[IBIS Ver]   4.0
[Comment Char] |_char
[File name]   pse84_wlb154.ibs
[File Rev] 1.2
[Date] 10/27/2023
[Source] Infineon Technologies IBIS team
[Notes]
|Rev. 1.0 - Initial model 12/8/2021
|Rev. 1.1 - Update with RLC 8/17/2023
|Rev. 1.2 - Included pins for MIPI-DPHY DSI and USB 10/23/2023
|Supports 1.8 V IO Interface and 3.3 V RF Switch Control Interface.
|The temperature range is -40 to 125C.
|This model was syntax checked with Hyperlynx 4.2 visual IBIS
|editor and ibischk7_64 IBIS checker.
|There were 0 syntax errors.
[Disclaimer]   The model given below represents a 220-pin package.
[Copyright]   (C) COPYRIGHT 2023, Infineon Technologies AG.
[Component] PSOCE84
[Manufacturer] Infineon Technologies AG
| Package model WLBGA154 was extracted from simulation tool.
[Package]
|   typ   min   max
R_pkg   0.37778   0.02885   0.99963
L_pkg   0.755n   0.113n   1.94n
C_pkg   0.272p   0.0783p   0.61p
[Pin]   Signal_name   model_name   R_pin   L_pin   C_pin
|L5   DSI_CLK_N_PAD   PAD   0.18036 3.56E-10   1.32E-13
|L4   DSI_CLK_P_PAD   PAD   0.22925 5.05E-10   1.68E-13
|J5   DSI_DATA0_N_PAD PAD   0.34681 7.02E-10   1.90E-13
|H5   DSI_DATA0_P_PAD PAD   0.32737 6.89E-10   1.82E-13
|H4   DSI_DATA1_N_PAD PAD   0.35927 7.29E-10   1.94E-13
|J4   DSI_DATA1_P_PAD PAD   0.34002 6.83E-10   1.82E-13
|G5   DSI_REXT_PAD   PAD   0.17871 5.97E-10   3.09E-13
G4   P12_0_PAD   1p8_ioi2c_wbso_h   0.58601 1.03E-09   3.09E-13
F5   P12_1_PAD   1p8_ioi2c_wbso_h   0.66384 1.24E-09   3.42E-13
F6   P12_2_PAD   1p8_ioi2c_wbso_h   0.76369 1.39E-09   4.00E-13
F7   P12_3_PAD   1p8_ioi2c_wbso_h   0.81887 1.50E-09   4.18E-13
F8   P12_4_PAD   1p8_ioi2c_wbso_h   0.93099 1.68E-09   5.32E-13
F9   P12_5_PAD   1p8_ioi2c_wbso_h   0.99963 1.80E-09   5.79E-13
G14   P13_0_PAD   1p8_gpib_3swbso_h   0.065427 1.91E-10   1.40E-13
J14   P13_1_PAD   1p8_ioi2c_wbso_h   0.29198 5.62E-10   1.54E-13
F14   P13_2_PAD   1p8_ioi2c_wbso_h   0.028854 1.35E-10   1.02E-13
K14   P13_3_PAD   1p8_ioi2c_wbso_h   0.39961 7.26E-10   3.44E-13
K13   P13_4_PAD   1p8_ioi2c_wbso_h   0.42314 7.99E-10   3.99E-13
E14   P13_5_PAD   1p8_gpib_3swbso_h   0.042433 1.13E-10   2.05E-13
G13   P14_3_PAD   1p8_ioi2c_wbso_h   0.32481 6.11E-10   2.16E-13
J13   P14_4_PAD   1p8_ioi2c_wbso_h   0.4981  8.90E-10   2.78E-13
C14   P15_0_PAD   1p8_ioi2c_wbso_h   0.14092 3.40E-10   1.43E-13
B14   P15_1_PAD   1p8_ioi2c_wbso_h   0.050643 2.09E-10   1.07E-13
G12   P15_2_PAD   1p8_ioi2c_wbso_h   0.55579 1.00E-09   4.33E-13
D13   P15_3_PAD   1p8_ioi2c_wbso_h   0.27529 5.42E-10   1.89E-13
J12   P16_0_PAD   3p3_gpio_wbso_h 0.77613 1.26E-09   5.75E-13
H11   P16_1_PAD   3p3_gpio_wbso_h 0.6983  1.20E-09   4.40E-13
A12   P16_2_PAD   3p3_gpio_wbso_h 0.039971   1.63E-10   9.91E-14
G11   P16_3_PAD   3p3_gpio_wbso_h 0.62882 1.11E-09   3.34E-13
F11   P16_4_PAD   3p3_gpio_wbso_h 0.53345 9.60E-10   3.01E-13
E11   P16_5_PAD   3p3_gpio_wbso_h 0.43008 8.36E-10   2.56E-13
D11   P16_6_PAD   3p3_gpio_wbso_h 0.31519 7.16E-10   2.19E-13
A11   P16_7_PAD   3p3_gpio_wbso_h 0.064   2.05E-10   1.16E-13
G10   P17_0_PAD   3p3_gpio_wbso_h 0.57169 1.07E-09   4.73E-13
F10   P17_1_PAD   3p3_gpio_wbso_h 0.51457 9.91E-10   2.90E-13
E10   P17_2_PAD   3p3_gpio_wbso_h 0.40617 8.30E-10   2.58E-13
E9   P17_3_PAD   3p3_gpio_wbso_h 0.42474 8.38E-10   2.51E-13
D10   P17_4_PAD   3p3_gpio_wbso_h 0.36553 7.76E-10   2.34E-13
D9   P17_5_PAD   3p3_gpio_wbso_h 0.36885 7.43E-10   2.30E-13
C10   P17_6_PAD   3p3_gpio_wbso_h 0.31893 7.04E-10   2.20E-13
H7   P18_0_PAD   1p8_gpib_3swbso_h   0.35662 6.76E-10   2.25E-13
J7   P18_1_PAD   1p8_gpib_3swbso_h   0.25345 4.81E-10   1.87E-13
G8   P19_0_PAD   1p8_gpib_3swbso_h   0.44499 8.18E-10   2.58E-13
H8   P19_1_PAD   1p8_gpib_3swbso_h   0.35458 6.30E-10   2.94E-13
A10   P2_0_PAD   1p8_hsio_wbso_h   0.53479 1.94E-09   6.10E-13
F4   P21_0_PAD   1p8_ioi2c_wbso_h   0.62566 1.14E-09   3.26E-13
E6   P21_1_PAD   1p8_ioi2c_wbso_h   0.67341 1.49E-09   5.08E-13
E5   P21_2_PAD   1p8_ioi2c_wbso_h   0.71959 1.27E-09   5.11E-13
E4   P21_3_PAD   1p8_ioi2c_wbso_h   0.69725 1.16E-09   4.87E-13
D6   P21_7_PAD   1p8_ioi2c_wbso_h   0.54873 1.61E-09   4.24E-13
E7   P3_0_PAD   1p8_ioi3c_3swbso_h   0.61597 1.16E-09   4.22E-13
E8   P3_1_PAD   1p8_ioi3c_3swbso_h   0.71724 1.31E-09   4.44E-13
D5   P5_0_PAD   1p8_hsio_wbso_h   0.42028 8.07E-10   3.21E-13
A7   P6_0_PAD   1p8_ioi2c_wbso_h   0.55769 1.01E-09   2.67E-13
A8   P6_1_PAD   1p8_ioi2c_wbso_h   0.64657 1.13E-09   3.81E-13
A9   P6_2_PAD   1p8_ioi2c_wbso_h   0.74835 1.30E-09   4.11E-13
B9   P6_3_PAD   1p8_ioi2c_wbso_h   0.80638 1.39E-09   3.80E-13
B8   P6_4_PAD   1p8_ioi2c_wbso_h   0.68861 1.23E-09   3.71E-13
B7   P6_5_PAD   1p8_ioi2c_wbso_h   0.56908 1.09E-09   3.03E-13
B6   P6_6_PAD   1p8_ioi2c_wbso_h   0.49405 9.55E-10   2.74E-13
B5   P6_7_PAD   1p8_ioi2c_wbso_h   0.4033  7.67E-10   2.41E-13
B4   P7_0_PAD   1p8_ioi2c_wbso_h   0.33297 6.49E-10   2.14E-13
C9   P7_1_PAD   1p8_ioi2c_wbso_h   0.75055 1.38E-09   3.65E-13
C8   P7_2_PAD   1p8_ioi2c_wbso_h   0.66864 1.24E-09   3.53E-13
C7   P7_3_PAD   1p8_ioi2c_wbso_h   0.57537 1.10E-09   3.07E-13
C6   P7_4_PAD   1p8_ioi2c_wbso_h   0.49102 9.49E-10   2.74E-13
C5   P7_5_PAD   1p8_ioi2c_wbso_h   0.39395 7.72E-10   2.39E-13
D8   P7_6_PAD   1p8_ioi2c_wbso_h   0.67974 1.27E-09   3.45E-13
D7   P7_7_PAD   1p8_ioi2c_wbso_h   0.60153 1.13E-09   3.19E-13
G9   P8_0_PAD   1p8_ioi2c_wbso_h   0.56702 1.05E-09   3.97E-13
G7   P8_1_PAD   1p8_ioi2c_wbso_h   0.4223  8.34E-10   2.53E-13
G6   P8_2_PAD   1p8_ioi2c_wbso_h   0.42072 7.87E-10   2.48E-13
H6   P8_3_PAD   1p8_ioi2c_wbso_h   0.33612 6.35E-10   2.20E-13
J6   P8_4_PAD   1p8_ioi2c_wbso_h   0.24079 4.88E-10   1.82E-13
A14   P9_0_PAD   1p8_ioi2c_wbso_h   0.072654 2.78E-10   1.15E-13
C13   P9_1_PAD   1p8_ioi2c_wbso_h   0.27424 5.46E-10   1.40E-13
B13   P9_2_PAD   1p8_ioi2c_wbso_h   0.168   3.82E-10   1.51E-13
A13   P9_3_PAD   1p8_ioi2c_wbso_h   0.072792 2.45E-10   2.53E-13
B3   SMIF0_SPIHB_CLK_P_PAD   Mpad_1   0.15376 4.98E-10   2.36E-13
B1   SMIF0_SPIHB_DATA0_PAD   Mpad   0.06842 2.50E-10   1.42E-13
B2   SMIF0_SPIHB_DATA1_PAD   Mpad   0.26384 4.40E-10   1.72E-13
C1   SMIF0_SPIHB_DATA2_PAD   Mpad   0.099463   2.76E-10   2.45E-13
C2   SMIF0_SPIHB_DATA3_PAD   Mpad   0.087686   2.79E-10   1.97E-13
D3   SMIF0_SPIHB_DATA4_PAD   Mpad   0.13026 3.54E-10   2.32E-13
D1   SMIF0_SPIHB_DATA5_PAD   Mpad   0.10161 2.70E-10   1.51E-13
E1   SMIF0_SPIHB_DATA6_PAD   Mpad   0.053124   2.27E-10   1.27E-13
D2   SMIF0_SPIHB_DATA7_PAD   Mpad   0.11769 3.42E-10   3.11E-13
E2   SMIF0_SPIHB_RWDS_PAD   Mpad   0.073654   2.41E-10   1.35E-13
H2   SMIF1_SPIHB_CLK_P_PAD   Mpad_1   0.09509 2.84E-10   2.92E-13
K1   SMIF1_SPIHB_DATA0_PAD   Mpad   0.092716   2.70E-10   1.56E-13
K2   SMIF1_SPIHB_DATA1_PAD   Mpad   0.088476   2.85E-10   1.65E-13
J1   SMIF1_SPIHB_DATA2_PAD   Mpad   0.043386   1.95E-10   1.19E-13
J2   SMIF1_SPIHB_DATA3_PAD   Mpad   0.083757   2.60E-10   2.70E-13
H1   SMIF1_SPIHB_DATA4_PAD   Mpad   0.04767 1.96E-10   7.83E-14
G2   SMIF1_SPIHB_DATA5_PAD   Mpad   0.12791 3.06E-10   2.33E-13
G1   SMIF1_SPIHB_DATA6_PAD   Mpad   0.05307 2.39E-10   1.38E-13
F2   SMIF1_SPIHB_DATA7_PAD   Mpad   0.077603   3.03E-10   1.72E-13
F1   SMIF1_SPIHB_RWDS_PAD   Mpad   0.03231 2.02E-10   1.17E-13
|A6   USB_DM_PAD   PAD   0.33189 7.32E-10   2.53E-13
|A5   USB_DP_PAD   PAD   0.29289 5.76E-10   2.42E-13
F3   VCCD_0_PAD   POWER
H14   VCCD_1_PAD   POWER
J9   VCCD_2_PAD   POWER
A4   VCCD_3_PAD   POWER
L1   VCCD_4_PAD   POWER
K9   VCCD_ANA_PAD   POWER
K12   VCCI_SR1P8_0_PAD   POWER
L10   VCCIRETLDO_PAD  POWER
J10   VCCRET_PAD   POWER
H10   VCCSRAM_PAD   POWER
H12   VCCSRAMI_0_PAD  POWER
C4   VCCSRAMI_1_PAD  POWER
A2   VDD33_USB_PAD   POWER
F12   VDDA_PAD   POWER
G3   VDDD_DLL_PAD   POWER
L8   VDDD_PAD   POWER
L12   VDDD_SR1P8_PAD  POWER
L9   VDDDLDO_PAD   POWER
A1   VDDIO_0_PAD   POWER
L6   VDDIO_1_PAD   POWER
B10   VDDIO_1P8_3P3_PAD   POWER
B12   VDDIO_2_PAD   POWER
L3   VDDIO_4_PAD   POWER
F13   VDDIO_A_PAD   POWER
D12   VDDIO_A_Q_PAD   POWER
J8   VDDIO_CO_PAD   POWER
C3   VDDIO_SMIF0_0_PAD   POWER
D4   VDDIO_SMIF0_1_PAD   POWER
K3   VDDIO_SMIF1_0_PAD   POWER
H3   VDDIO_SMIF1_1_PAD   POWER
L13   VDDLX_SR1P8_PAD POWER
C11   VDDP_PAD   POWER
L7   VDDPUMP_RRAM_PAD   POWER
K11   VDDQ_0_PAD   POWER
L11   VDDQ_SR1P8_PAD  POWER
K5   VP_DSI_PAD   POWER
K6   VPH_P_DSI_PAD   POWER
D14   VREF_PAD   POWER
L14   VSS_SR1P8_PAD   GND
C12   VSSA0   GND
E12   VSSA1   GND
E13   VSSA2   GND
A3   VSSD   GND
B11   VSSD   GND
E3   VSSD   GND
H13   VSSD   GND
J3   VSSD   GND
K4   VSSD   GND
K7   VSSD   GND
K8   VSSD   GND
L2   VSSD   GND
J11   VSSQ_PAD   GND
K10   VSSQ_PAD   GND
H9   XRES_PAD   1p8_xres_3swbso 0.4163  7.27E-10   3.26E-13
|   MODEL SELECTOR
[Model Selector] 1p8_hsio_wbso_h
| Model Description
hsio_drive000_slew0  obuf mode with drive_sel=000 and slew_sel=0
hsio_drive000_slew1  obuf mode with drive_sel=000 and slew_sel=1
hsio_drive001_slew0  obuf mode with drive_sel=001 and slew_sel=0
hsio_drive001_slew1  obuf mode with drive_sel=001 and slew_sel=1
hsio_drive010_slew0  obuf mode with drive_sel=010 and slew_sel=0
hsio_drive010_slew1  obuf mode with drive_sel=010 and slew_sel=1
hsio_drive011_slew0  obuf mode with drive_sel=011 and slew_sel=0
hsio_drive011_slew1  obuf mode with drive_sel=011 and slew_sel=1
hsio_drive100_slew0  obuf mode with drive_sel=100 and slew_sel=0
hsio_drive100_slew1  obuf mode with drive_sel=100 and slew_sel=1
hsio_drive101_slew0  obuf mode with drive_sel=101 and slew_sel=0
hsio_drive101_slew1  obuf mode with drive_sel=101 and slew_sel=1
hsio_drive110_slew0  obuf mode with drive_sel=110 and slew_sel=0
hsio_drive110_slew1  obuf mode with drive_sel=110 and slew_sel=1
hsio_drive111_slew0  obuf mode with drive_sel=111 and slew_sel=0
hsio_drive111_slew1  obuf mode with drive_sel=111 and slew_sel=1
[Model Selector] 1p8_ioi2c_wbso_h
| Model Description
ioi2c_drive000_slew0   obuf mode with drive_sel=000 and slew_sel=0
ioi2c_drive000_slew1   obuf mode with drive_sel=000 and slew_sel=1
ioi2c_drive100_slew0   obuf mode with drive_sel=100 and slew_sel=0
ioi2c_drive100_slew1   obuf mode with drive_sel=100 and slew_sel=1
ioi2c_drive010_slew0   obuf mode with drive_sel=010 and slew_sel=0
ioi2c_drive010_slew1   obuf mode with drive_sel=010 and slew_sel=1
ioi2c_drive110_slew0   obuf mode with drive_sel=110 and slew_sel=0
ioi2c_drive110_slew1   obuf mode with drive_sel=110 and slew_sel=1
ioi2c_drive001_slew0   obuf mode with drive_sel=001 and slew_sel=0
ioi2c_drive001_slew1   obuf mode with drive_sel=001 and slew_sel=1
ioi2c_drive101_slew0   obuf mode with drive_sel=101 and slew_sel=0
ioi2c_drive101_slew1   obuf mode with drive_sel=101 and slew_sel=1
ioi2c_drive011_slew0   obuf mode with drive_sel=011 and slew_sel=0
ioi2c_drive011_slew1   obuf mode with drive_sel=011 and slew_sel=1
ioi2c_drive111_slew0   obuf mode with drive_sel=111 and slew_sel=0
ioi2c_drive111_slew1   obuf mode with drive_sel=111 and slew_sel=1
ioi2c_drive000_slow1   obuf mode with drive_sel=000 and slow=1
ioi2c_drive100_slow1   obuf mode with drive_sel=100 and slow=1
ioi2c_drive010_slow1   obuf mode with drive_sel=010 and slow=1
ioi2c_drive110_slow1   obuf mode with drive_sel=110 and slow=1
ioi2c_drive001_slow1   obuf mode with drive_sel=001 and slow=1
ioi2c_drive101_slow1   obuf mode with drive_sel=101 and slow=1
ioi2c_drive011_slow1   obuf mode with drive_sel=011 and slow=1
ioi2c_drive111_slow1   obuf mode with drive_sel=111 and slow=1
[Model Selector] 1p8_ioi3c_3swbso_h
| Model Description
ioi3c_drive000_slew0   obuf mode with drive_sel=000 and slew_sel=0
ioi3c_drive000_slew1   obuf mode with drive_sel=000 and slew_sel=1
ioi3c_drive100_slew0   obuf mode with drive_sel=100 and slew_sel=0
ioi3c_drive100_slew1   obuf mode with drive_sel=100 and slew_sel=1
ioi3c_drive010_slew0   obuf mode with drive_sel=010 and slew_sel=0
ioi3c_drive010_slew1   obuf mode with drive_sel=010 and slew_sel=1
ioi3c_drive110_slew0   obuf mode with drive_sel=110 and slew_sel=0
ioi3c_drive110_slew1   obuf mode with drive_sel=110 and slew_sel=1
ioi3c_drive001_slew0   obuf mode with drive_sel=001 and slew_sel=0
ioi3c_drive001_slew1   obuf mode with drive_sel=001 and slew_sel=1
ioi3c_drive101_slew0   obuf mode with drive_sel=101 and slew_sel=0
ioi3c_drive101_slew1   obuf mode with drive_sel=101 and slew_sel=1
ioi3c_drive011_slew0   obuf mode with drive_sel=011 and slew_sel=0
ioi3c_drive011_slew1   obuf mode with drive_sel=011 and slew_sel=1
ioi3c_drive111_slew0   obuf mode with drive_sel=111 and slew_sel=0
ioi3c_drive111_slew1   obuf mode with drive_sel=111 and slew_sel=1
ioi3c_drive000_slow1   obuf mode with drive_sel=000 and slow=1
ioi3c_drive100_slow1   obuf mode with drive_sel=100 and slow=1
ioi3c_drive010_slow1   obuf mode with drive_sel=010 and slow=1
ioi3c_drive110_slow1   obuf mode with drive_sel=110 and slow=1
ioi3c_drive001_slow1   obuf mode with drive_sel=001 and slow=1
ioi3c_drive101_slow1   obuf mode with drive_sel=101 and slow=1
ioi3c_drive011_slow1   obuf mode with drive_sel=011 and slow=1
ioi3c_drive111_slow1   obuf mode with drive_sel=111 and slow=1
[Model Selector] 3p3_gpio_wbso_h
| Model Description
gpio_000_slew0_slow0   obuf mode with drive_sel=000 and slew_sel=0
gpio_000_slew1_slow0   obuf mode with drive_sel=000 and slew_sel=1
gpio_100_slew0_slow0   obuf mode with drive_sel=100 and slew_sel=0
gpio_100_slew1_slow0   obuf mode with drive_sel=100 and slew_sel=1
gpio_010_slew0_slow0   obuf mode with drive_sel=010 and slew_sel=0
gpio_010_slew1_slow0   obuf mode with drive_sel=010 and slew_sel=1
gpio_110_slew0_slow0   obuf mode with drive_sel=110 and slew_sel=0
gpio_110_slew1_slow0   obuf mode with drive_sel=110 and slew_sel=1
gpio_001_slew0_slow0   obuf mode with drive_sel=001 and slew_sel=0
gpio_001_slew1_slow0   obuf mode with drive_sel=001 and slew_sel=1
gpio_101_slew0_slow0   obuf mode with drive_sel=101 and slew_sel=0
gpio_101_slew1_slow0   obuf mode with drive_sel=101 and slew_sel=1
gpio_011_slew0_slow0   obuf mode with drive_sel=011 and slew_sel=0
gpio_011_slew1_slow0   obuf mode with drive_sel=011 and slew_sel=1
gpio_111_slew0_slow0   obuf mode with drive_sel=111 and slew_sel=0
gpio_111_slew1_slow0   obuf mode with drive_sel=111 and slew_sel=1
gpio_000_slew0_slow1   obuf mode with drive_sel=000 for slow=1 and slew=0
gpio_000_slew1_slow1   obuf mode with drive_sel=000 for slow=1 and slew=1
gpio_100_slew0_slow1   obuf mode with drive_sel=100 for slow=1 and slew=0
gpio_100_slew1_slow1   obuf mode with drive_sel=100 for slow=1 and slew=1
gpio_010_slew0_slow1   obuf mode with drive_sel=010 for slow=1 and slew=0
gpio_010_slew1_slow1   obuf mode with drive_sel=010 for slow=1 and slew=1
gpio_110_slew0_slow1   obuf mode with drive_sel=110 for slow=1 and slew=0
gpio_110_slew1_slow1   obuf mode with drive_sel=110 for slow=1 and slew=1
gpio_001_slew0_slow1   obuf mode with drive_sel=001 for slow=1 and slew=0
gpio_001_slew1_slow1   obuf mode with drive_sel=001 for slow=1 and slew=1
gpio_101_slew0_slow1   obuf mode with drive_sel=101 for slow=1 and slew=0
gpio_101_slew1_slow1   obuf mode with drive_sel=101 for slow=1 and slew=1
gpio_011_slew0_slow1   obuf mode with drive_sel=011 for slow=1 and slew=0
gpio_011_slew1_slow1   obuf mode with drive_sel=011 for slow=1 and slew=1
gpio_111_slew0_slow1   obuf mode with drive_sel=111 for slow=1 and slew=0
gpio_111_slew1_slow1   obuf mode with drive_sel=111 for slow=1 and slew=1
| pad
[Model Selector] Mpad
| Model Description
hsio_drive000_slew0  obuf mode with drive_sel=000 and slew_sel=0
hsio_drive000_slew1  obuf mode with drive_sel=000 and slew_sel=1
hsio_drive001_slew0  obuf mode with drive_sel=001 and slew_sel=0
hsio_drive001_slew1  obuf mode with drive_sel=001 and slew_sel=1
hsio_drive010_slew0  obuf mode with drive_sel=010 and slew_sel=0
hsio_drive010_slew1  obuf mode with drive_sel=010 and slew_sel=1
hsio_drive011_slew0  obuf mode with drive_sel=011 and slew_sel=0
hsio_drive011_slew1  obuf mode with drive_sel=011 and slew_sel=1
hsio_drive100_slew0  obuf mode with drive_sel=100 and slew_sel=0
hsio_drive100_slew1  obuf mode with drive_sel=100 and slew_sel=1
hsio_drive101_slew0  obuf mode with drive_sel=101 and slew_sel=0
hsio_drive101_slew1  obuf mode with drive_sel=101 and slew_sel=1
hsio_drive110_slew0  obuf mode with drive_sel=110 and slew_sel=0
hsio_drive110_slew1  obuf mode with drive_sel=110 and slew_sel=1
hsio_drive111_slew0  obuf mode with drive_sel=111 and slew_sel=0
hsio_drive111_slew1  obuf mode with drive_sel=111 and slew_sel=1
[Model Selector] Mpad_1
| Model Description
p1_drive000_slew0  obuf mode with drive_sel=000 and slew_sel=0
p1_drive000_slew1  obuf mode with drive_sel=000 and slew_sel=1
p1_drive001_slew0  obuf mode with drive_sel=001 and slew_sel=0
p1_drive001_slew1  obuf mode with drive_sel=001 and slew_sel=1
p1_drive010_slew0  obuf mode with drive_sel=010 and slew_sel=0
p1_drive010_slew1  obuf mode with drive_sel=010 and slew_sel=1
p1_drive011_slew0  obuf mode with drive_sel=011 and slew_sel=0
p1_drive011_slew1  obuf mode with drive_sel=011 and slew_sel=1
p1_drive100_slew0  obuf mode with drive_sel=100 and slew_sel=0
p1_drive100_slew1  obuf mode with drive_sel=100 and slew_sel=1
p1_drive101_slew0  obuf mode with drive_sel=101 and slew_sel=0
p1_drive101_slew1  obuf mode with drive_sel=101 and slew_sel=1
p1_drive110_slew0  obuf mode with drive_sel=110 and slew_sel=0
p1_drive110_slew1  obuf mode with drive_sel=110 and slew_sel=1
p1_drive111_slew0  obuf mode with drive_sel=111 and slew_sel=0
p1_drive111_slew1  obuf mode with drive_sel=111 and slew_sel=1
| Models and submodels in the file (114): 1p8_gpib_3swbso_h (Input), ioi2c_drive000_slew0 (I/O), ioi2c_drive000_slew1 (I/O), ioi2c_drive100_slew0 (I/O), ioi2c_drive100_slew1 (I/O), ioi2c_drive010_slew0 (I/O), ioi2c_drive010_slew1 (I/O), ioi2c_drive110_slew0 (I/O), ioi2c_drive110_slew1 (I/O), ioi2c_drive001_slew0 (I/O), ioi2c_drive001_slew1 (I/O), ioi2c_drive101_slew0 (I/O), ioi2c_drive101_slew1 (I/O), ioi2c_drive011_slew0 (I/O), ioi2c_drive011_slew1 (I/O), ioi2c_drive111_slew0 (I/O), ioi2c_drive111_slew1 (I/O), ioi2c_drive000_slow1 (I/O), ioi2c_drive100_slow1 (I/O), ioi2c_drive010_slow1 (I/O), ioi2c_drive110_slow1 (I/O), ioi2c_drive001_slow1 (I/O), ioi2c_drive101_slow1 (I/O), ioi2c_drive011_slow1 (I/O), ioi2c_drive111_slow1 (I/O), ioi3c_drive000_slew0 (I/O), ioi3c_drive000_slew1 (I/O), ioi3c_drive100_slew0 (I/O), ioi3c_drive100_slew1 (I/O), ioi3c_drive010_slew0 (I/O), ioi3c_drive010_slew1 (I/O), ioi3c_drive110_slew0 (I/O), ioi3c_drive110_slew1 (I/O), ioi3c_drive001_slew0 (I/O), ioi3c_drive001_slew1 (I/O), ioi3c_drive101_slew0 (I/O), ioi3c_drive101_slew1 (I/O), ioi3c_drive011_slew0 (I/O), ioi3c_drive011_slew1 (I/O), ioi3c_drive111_slew0 (I/O), ioi3c_drive111_slew1 (I/O), ioi3c_drive000_slow1 (I/O), ioi3c_drive100_slow1 (I/O), ioi3c_drive010_slow1 (I/O), ioi3c_drive110_slow1 (I/O), ioi3c_drive001_slow1 (I/O), ioi3c_drive101_slow1 (I/O), ioi3c_drive011_slow1 (I/O), ioi3c_drive111_slow1 (I/O), 1p8_xres_3swbso (Input), gpio_000_slew0_slow0 (I/O), gpio_000_slew1_slow0 (I/O), gpio_100_slew0_slow0 (I/O), gpio_100_slew1_slow0 (I/O), gpio_010_slew0_slow0 (I/O), gpio_010_slew1_slow0 (I/O), gpio_110_slew0_slow0 (I/O), gpio_110_slew1_slow0 (I/O), gpio_001_slew0_slow0 (I/O), gpio_001_slew1_slow0 (I/O), gpio_101_slew0_slow0 (I/O), gpio_101_slew1_slow0 (I/O), gpio_011_slew0_slow0 (I/O), gpio_011_slew1_slow0 (I/O), gpio_111_slew0_slow0 (I/O), gpio_111_slew1_slow0 (I/O), gpio_000_slew0_slow1 (I/O), gpio_000_slew1_slow1 (I/O), gpio_100_slew0_slow1 (I/O), gpio_100_slew1_slow1 (I/O), gpio_010_slew0_slow1 (I/O), gpio_010_slew1_slow1 (I/O), gpio_110_slew0_slow1 (I/O), gpio_110_slew1_slow1 (I/O), gpio_001_slew0_slow1 (I/O), gpio_001_slew1_slow1 (I/O), gpio_101_slew0_slow1 (I/O), gpio_101_slew1_slow1 (I/O), gpio_011_slew0_slow1 (I/O), gpio_011_slew1_slow1 (I/O)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
